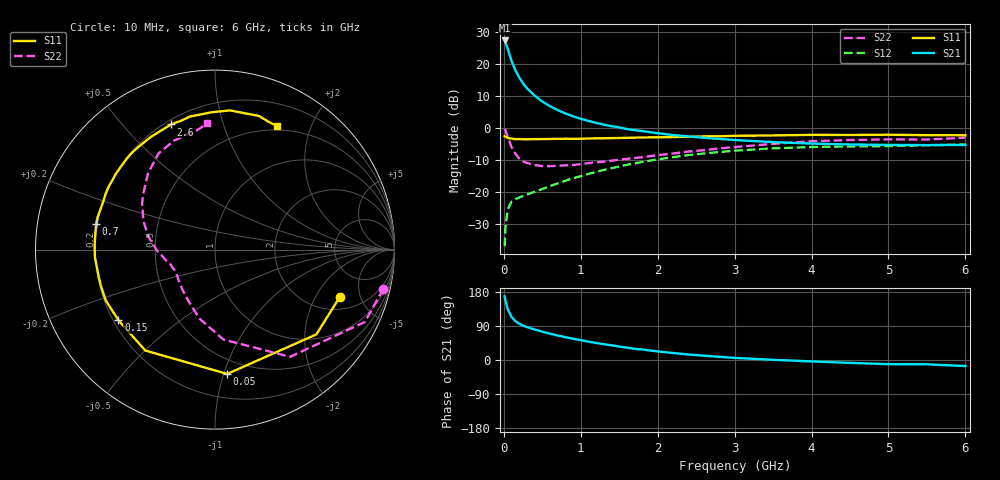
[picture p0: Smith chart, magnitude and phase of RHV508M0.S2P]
! SIEMENS Small Signal Semiconductors
! BFR106
! Si NPN RF Bipolar Junction Transistor in SOT23
! VCE = 0.5 V  IC = 8 mA
! Common Emitter S-Parameters:  August  1996
# GHz  S  MA  R  50
!  f  S11  S21  S12  S22
! GHz  MAG  ANG  MAG  ANG  MAG  ANG  MAG  ANG
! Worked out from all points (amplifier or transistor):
!   36 points, 10 MHz to 6 GHz, reference 50 ohm
!   highest |S21| = 27.4 dB at 10 MHz (marker M1)
!   |S21| within 3 dB of that: start of sweep to 54.42 MHz
!   unconditionally stable (mu >= 1): 471.5 MHz to end of sweep
!   at 250 MHz: K = 0.68, MSG = 17.6 dB, |S12| = -21.3 dB
!   at 1.4 GHz: K = 1.16, MAG = 4.1 dB, |S12| = -12.6 dB
!   at 6 GHz: K = 1.03, MAG = -1.2 dB, |S12| = -5.2 dB
!   S11 on the Smith chart (normalised r, x): 10 MHz: 2.78, -3.26; 50 MHz: 0.38, -1.03; 150 MHz: 0.22, -0.31; 700 MHz: 0.19, +0.10; 2.6 GHz: 0.22, +0.69; 6 GHz: 0.45, +1.52
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0.01  0.7441 -20.6  23.5 168.2  0.0141 81.3  0.9637 -13.1
0.02  0.7365 -39.9  22.44 158.3  0.0269 72.0  0.9269 -25.8
0.05  0.6959 -84.4  17.28 134.2  0.0532 52.0  0.7293 -55.0
0.1  0.6833 -124.6  11.27 113.5  0.0703 38.2  0.503 -84.7
0.15  0.6669 -143.8  7.992 102.5  0.0769 33.9  0.3949 -102.5
0.2  0.6715 -155.2  6.196 95.8  0.0818 34.1  0.334 -114.2
0.25  0.667 -162.7  4.995 90.5  0.0861 34.8  0.3002 -124.3
0.3  0.6652 -167.9  4.201 86.9  0.0906 36.4  0.2836 -130.7
0.4  0.6701 -176.2  3.212 80.4  0.1003 40.0  0.2626 -141.2
0.5  0.6712 178.1  2.595 74.8  0.1109 42.9  0.2535 -148.2
0.6  0.6729 172.4  2.191 69.4  0.1232 45.3  0.2525 -152.7
0.7  0.677 167.7  1.907 64.6  0.1355 47.2  0.2564 -156.4
0.9  0.6761 160.3  1.527 56.1  0.1631 49.2  0.2633 -163.4
1.1  0.6849 152.6  1.292 48.4  0.1909 49.7  0.2816 -168.1
1.3  0.6901 145.8  1.129 41.7  0.2204 48.9  0.2973 -173.4
1.6  0.7014 136.9  0.963 32.5  0.2647 46.7  0.3291 179.5
2.2  0.722 120.0  0.776 18.4  0.3499 39.0  0.3984 164.0
2.6  0.739 109.3  0.702 11.3  0.399 32.7  0.4494 153.4
3.5  0.7653 91.5  0.601 0.5  0.4798 18.1  0.565 131.4
4.5  0.7775 77.5  0.552 -7.6  0.5138 3.6  0.6479 110.9
5.5  0.7721 67.3  0.54 -11.4  0.537 -4.9  0.6605 100.9
6  0.7699 63.4  0.543 -16.0  0.5517 -11.1  0.7047 93.4
